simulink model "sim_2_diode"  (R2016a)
settings: Solver=VariableStepAuto  StartTime=0.0  StopTime=10.0  MaxStep=0.001  RelTol=1e-3
libraries: simulink x1

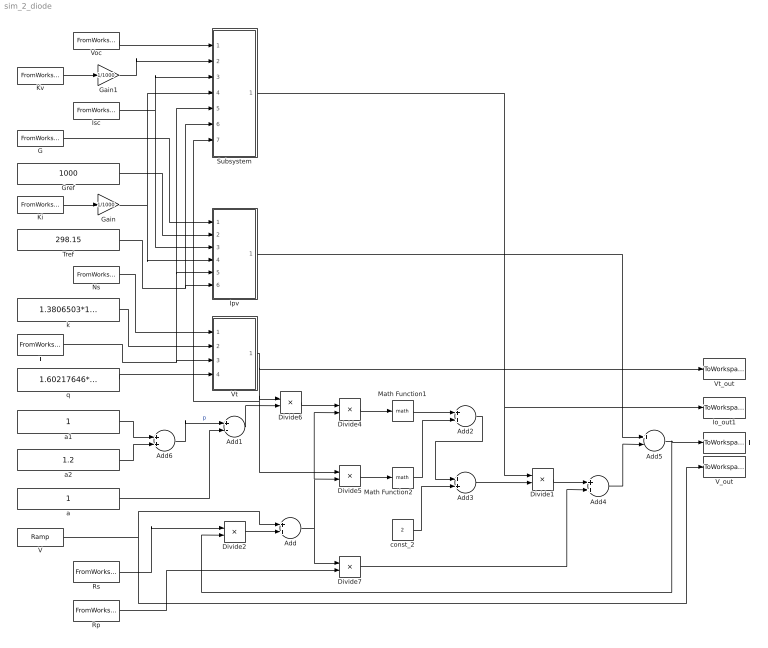
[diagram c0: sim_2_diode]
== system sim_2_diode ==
  Add{,2..4,6} (5 alike) : Sum
  Add1 : Sum  Inputs=+-
  Add5 : Sum  Inputs=+-
  Divide1 : Product  Inputs=**
  Divide2 : Product  Inputs=**
  Divide4 : Product  Inputs=/*
  Divide5 : Product  Inputs=/*
  Divide6 : Product  Inputs=**
  Divide7 : Product  Inputs=*/
  G : FromWorkspace  VariableName=G_in  SampleTime=0
  Gain : Gain  Gain=1/1000
  Gain1 : Gain  Gain=1/1000
  Gref : Constant  Value=1000
  I : ToWorkspace  VariableName=I_out  SaveFormat=Timeseries  SampleTime=-1
  Io_out1 : ToWorkspace  VariableName=Io_out  SaveFormat=Timeseries  SampleTime=-1
  Ipv : Subsystem
  Isc : FromWorkspace  VariableName=Isc_in  SampleTime=0
  Ki : FromWorkspace  VariableName=Ki_in  SampleTime=0
  Kv : FromWorkspace  VariableName=Kv_in  SampleTime=0
  Math Function1 : Math
  Math Function2 : Math
  Ns : FromWorkspace  VariableName=Ns_in  SampleTime=0
  Rp : FromWorkspace  VariableName=Rp_in  SampleTime=0
  Rs : FromWorkspace  VariableName=Rs_in  SampleTime=0
  Subsystem : Subsystem
  T : FromWorkspace  VariableName=T_in  SampleTime=0
  Tref : Constant  Value=298.15
  V : simulink/Sources/Ramp  slope=1  start=0  X0=0
  V_out : ToWorkspace  VariableName=V_out  SaveFormat=Timeseries  SampleTime=-1
  Voc : FromWorkspace  VariableName=Voc_in  SampleTime=0
  Vt : Subsystem
  Vt_out : ToWorkspace  VariableName=Vt_out  SaveFormat=Timeseries  SampleTime=-1
  a : Constant
  a1 : Constant
  a2 : Constant  Value=1.2
  const_2 : Constant  Value=2
  k : Constant  Value=1.3806503*10^-23
  q : Constant  Value=1.60217646*10^-19
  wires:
  Divide2/1 -> Add/2
  Rs/1 -> Divide2/1
  V/1 -> Add/1, V_out/1
  Divide4/1 -> Math Function1/1
  Divide5/1 -> Math Function2/1
  Add1/1 -> Divide6/2
  a/1 -> Add1/2
  Add/1 -> Divide7/1, Divide4/2, Divide5/2
  Divide6/1 -> Divide4/1
  Math Function1/1 -> Add2/1
  Math Function2/1 -> Add2/2
  Add2/1 -> Add3/1
  const_2/1 -> Add3/2
  Vt/1(Vt) -> Vt_out/1, Subsystem/7(Vt), Divide5/1, Divide6/1
  Ns/1 -> Vt/1(Ns)
  k/1 -> Vt/2(k)
  T/1 -> Vt/3(T), Ipv/5(T), Subsystem/5(T)
  q/1 -> Vt/4(q)
  G/1 -> Ipv/1(G)
  Gref/1 -> Ipv/2(Gref)
  Isc/1 -> Subsystem/3(Iscref), Ipv/3(Ipvref)
  Tref/1 -> Ipv/6(Tref), Subsystem/6(Tref)
  Rp/1 -> Divide7/2
  Add3/1 -> Divide1/2
  Divide7/1 -> Add4/2
  Divide1/1 -> Add4/1
  Add4/1 -> Add5/2
  Add5/1 -> I/1, Divide2/2
  Ipv/1(Ipv) -> Add5/1
  a1/1 -> Add6/1
  a2/1 -> Add6/2
  Add6/1 -> Add1/1  "p"
  Voc/1 -> Subsystem/1(Vocref)
  Subsystem/1(Io) -> Io_out1/1, Divide1/1
  Ki/1 -> Gain/1
  Gain/1 -> Ipv/4(Ksc), Subsystem/4(Ksc)
  Gain1/1 -> Subsystem/2(Kvo)
  Kv/1 -> Gain1/1

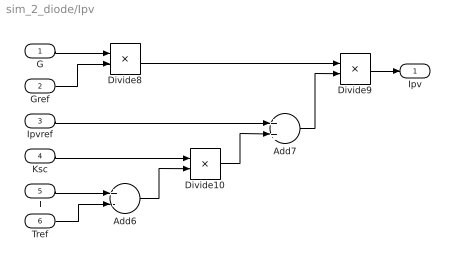
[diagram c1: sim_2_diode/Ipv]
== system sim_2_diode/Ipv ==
  G : Inport
  Gref : Inport  Port=2
  Ipvref : Inport  Port=3
  Ksc : Inport  Port=4
  T : Inport  Port=5
  Tref : Inport  Port=6
  Add6 : Sum  Inputs=+-
  Add7 : Sum
  Divide10 : Product  Inputs=**
  Divide8 : Product  Inputs=*/
  Divide9 : Product  Inputs=**
  Ipv : Outport
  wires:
  Divide9/1 -> Ipv/1
  T/1 -> Add6/1
  Divide8/1 -> Divide9/1
  Gref/1 -> Divide8/2
  G/1 -> Divide8/1
  Add7/1 -> Divide9/2
  Ksc/1 -> Divide10/1
  Add6/1 -> Divide10/2
  Ipvref/1 -> Add7/1
  Tref/1 -> Add6/2
  Divide10/1 -> Add7/2

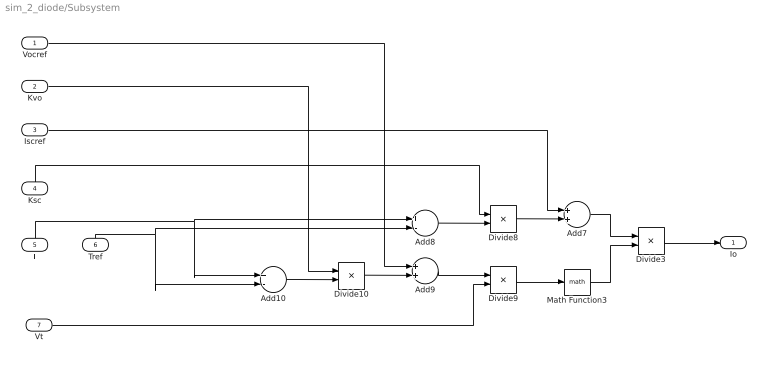
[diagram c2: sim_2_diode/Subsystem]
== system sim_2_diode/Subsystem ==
  Vocref : Inport
  Kvo : Inport  Port=2
  Iscref : Inport  Port=3
  Ksc : Inport  Port=4
  T : Inport  Port=5
  Tref : Inport  Port=6
  Vt : Inport  Port=7
  Add10 : Sum  Inputs=+-
  Add7 : Sum
  Add8 : Sum  Inputs=+-
  Add9 : Sum
  Divide10 : Product  Inputs=**
  Divide3 : Product  Inputs=*/
  Divide8 : Product  Inputs=**
  Divide9 : Product  Inputs=*/
  Math Function3 : Math
  Io : Outport
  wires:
  Add10/1 -> Divide10/2
  Add9/1 -> Divide9/1
  Divide10/1 -> Add9/2
  Divide8/1 -> Add7/2
  Vocref/1 -> Add9/1
  Add7/1 -> Divide3/1
  T/1 -> Add10/1, Add8/1
  Ksc/1 -> Divide8/1
  Tref/1 -> Add10/2, Add8/2
  Vt/1 -> Divide9/2
  Add8/1 -> Divide8/2
  Math Function3/1 -> Divide3/2
  Kvo/1 -> Divide10/1
  Divide3/1 -> Io/1
  Iscref/1 -> Add7/1
  Divide9/1 -> Math Function3/1

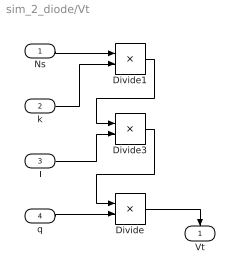
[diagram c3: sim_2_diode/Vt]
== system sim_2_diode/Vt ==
  Ns : Inport
  k : Inport  Port=2
  T : Inport  Port=3
  q : Inport  Port=4
  Divide : Product  Inputs=*/
  Divide1 : Product  Inputs=**
  Divide3 : Product  Inputs=**
  Vt : Outport
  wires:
  T/1 -> Divide3/2
  Ns/1 -> Divide1/1
  q/1 -> Divide/2
  Divide3/1 -> Divide/1
  Divide1/1 -> Divide3/1
  k/1 -> Divide1/2
  Divide/1 -> Vt/1
